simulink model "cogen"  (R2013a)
settings: Solver=ode45  StartTime=0.0  StopTime=24.0  RelTol=1e-3
libraries: simulink x2

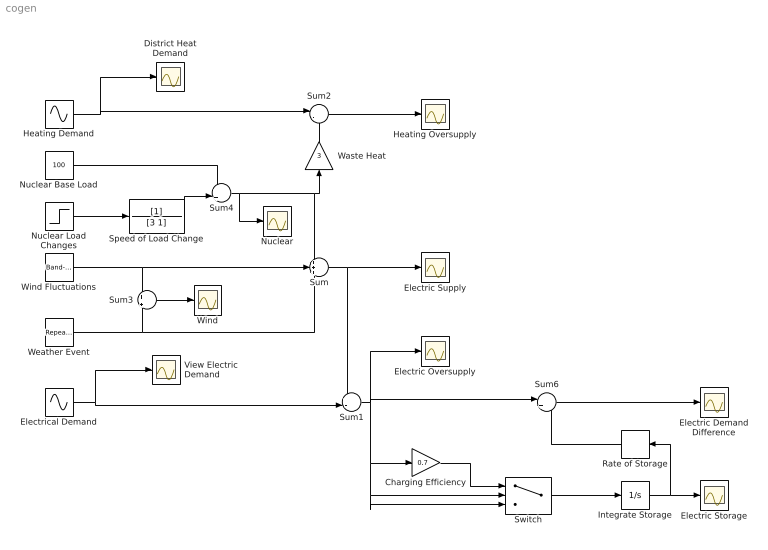
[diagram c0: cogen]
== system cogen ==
  Charging Efficiency : Gain  Gain=0.7
  District Heat Demand : Scope
  Electric Demand Difference : Scope
  Electric Oversupply : Scope
  Electric Storage : Scope
  Electric Supply : Scope
  Electrical Demand : Sin  Amplitude=30  Bias=80  Frequency=2*pi/24  Phase=1.3*pi  SampleTime=0
  Heating Demand : Sin  Amplitude=30  Bias=250  Frequency=2*pi/24  Phase=pi/2  SampleTime=0
  Heating Oversupply : Scope
  Integrate Storage : Integrator  LimitOutput=on  UpperSaturationLimit=200  LowerSaturationLimit=0
  Nuclear : Scope
  Nuclear Base Load : Constant  Value=100
  Nuclear Load Changes : Step  Time=1.0  After=-20  SampleTime=0
  Rate of Storage : Derivative
  Speed of Load Change : TransferFcn  Denominator=[3 1]
  Sum : Sum  Inputs=+++
  Sum1 : Sum  Inputs=+-|
  Sum2 : Sum  Inputs=|-+
  Sum3 : Sum  Inputs=+|+
  Sum4 : Sum  Inputs=+|+
  Sum6 : Sum  Inputs=|+-
  Switch : Switch
  View Electric Demand : Scope
  Waste Heat : Gain  Gain=3
  Weather Event : simulink/Sources/Repeating Sequence Stair  OutValues=[-1 -1 20 17 10 5 -1 -1].'  tsamp=1.5  OutMin=[]  OutMax=[]  OutDataTypeStr=double  OutputDataTypeScalingMode=double  OutDataType=fixdt(0,8)  ConRadixGroup=Best Precision: Vector-wise  OutScaling=2^-12
  Wind : Scope
  Wind Fluctuations : simulink/Sources/Band-Limited White Noise  Cov=[5]  Ts=0.5  seed=[23341]
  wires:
  Wind Fluctuations/1 -> Sum3/1, Sum/2
  Weather Event/1 -> Sum3/2, Sum/3
  Sum/1 -> Sum1/1, Electric Supply/1
  Sum1/1 -> Switch/3, Switch/2, Charging Efficiency/1, Sum6/1, Electric Oversupply/1
  Electrical Demand/1 -> View Electric Demand/1, Sum1/2
  Heating Demand/1 -> District Heat Demand/1, Sum2/1
  Sum2/1 -> Heating Oversupply/1
  Waste Heat/1 -> Sum2/2
  Nuclear Load Changes/1 -> Speed of Load Change/1
  Sum3/1 -> Wind/1
  Speed of Load Change/1 -> Sum4/2
  Nuclear Base Load/1 -> Sum4/1
  Sum4/1 -> Nuclear/1, Sum/1, Waste Heat/1
  Integrate Storage/1 -> Rate of Storage/1, Electric Storage/1
  Switch/1 -> Integrate Storage/1
  Rate of Storage/1 -> Sum6/2
  Sum6/1 -> Electric Demand Difference/1
  Charging Efficiency/1 -> Switch/1
